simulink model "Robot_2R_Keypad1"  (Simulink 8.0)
settings: Solver=ode3  StartTime=0.0  StopTime=inf  RelTol=1e-3
InitFcn:
  | dt=0.01;
  | Kp=400; Kd=0; Ki=0;
undefined symbols (not defined in the file or in its folder): DiscIntNeverNeededParam
libraries: arduinolib x9, simulink x2

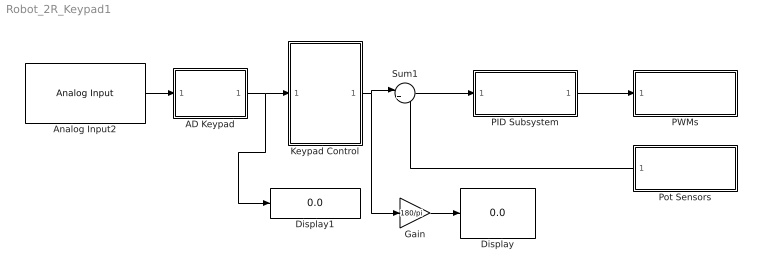
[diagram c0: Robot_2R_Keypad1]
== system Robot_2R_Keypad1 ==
  AD Keypad : MATLAB Function  TreatAsAtomicUnit=on
  Analog Input2 : arduinolib/Analog Input  pinNumber=2  sampleTime=dt
  Display : Display
  Display1 : Display
  Gain : Gain  Gain=180/pi
  Keypad Control : MATLAB Function  TreatAsAtomicUnit=on
  PID Subsystem : Subsystem  TreatAsAtomicUnit=on
  PWMs : Subsystem  TreatAsAtomicUnit=on
  Pot Sensors : Subsystem  TreatAsAtomicUnit=on
  Sum1 : Sum  Inputs=|+-
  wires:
  PID Subsystem/1(Out1) -> PWMs/1(In1)
  Sum1/1 -> PID Subsystem/1(In1)
  Pot Sensors/1(Out1) -> Sum1/2
  Analog Input2/1 -> AD Keypad/1(u)
  AD Keypad/1(y) -> Display1/1, Keypad Control/1(key)
  Keypad Control/1(thd) -> Gain/1, Sum1/1
  Gain/1 -> Display/1

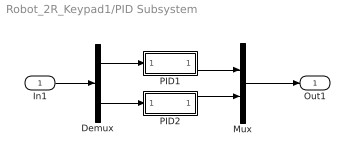
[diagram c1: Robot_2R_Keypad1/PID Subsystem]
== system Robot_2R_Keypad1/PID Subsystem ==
  In1 : Inport
  Demux : Demux  Outputs=2
  Mux : Mux  Inputs=2
  PID1 : Subsystem
  PID2 : Subsystem
  Out1 : Outport
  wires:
  In1/1 -> Demux/1
  Demux/1 -> PID1/1(In1)
  PID1/1(Out1) -> Mux/1
  Demux/2 -> PID2/1(In1)
  PID2/1(Out1) -> Mux/2
  Mux/1 -> Out1/1

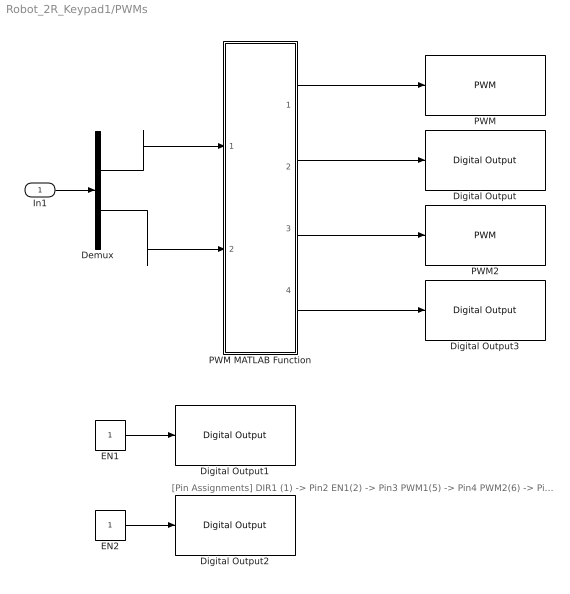
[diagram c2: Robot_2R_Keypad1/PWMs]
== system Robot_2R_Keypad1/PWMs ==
  note: [Pin Assignments] DIR1 (1) -> Pin2 EN1(2) -> Pin3 PWM1(5) -> Pin4 PWM2(6) -> Pin5 DIR2 (7) -> Pin6 EN2(8) -> Pin7
  In1 : Inport
  Demux : Demux  Outputs=2
  Digital Output : arduinolib/Digital Output  pinNumber=2
  Digital Output1 : arduinolib/Digital Output  pinNumber=3
  Digital Output2 : arduinolib/Digital Output  pinNumber=7
  Digital Output3 : arduinolib/Digital Output  pinNumber=6
  EN1 : Constant
  EN2 : Constant
  PWM : arduinolib/PWM  pinNumber=4
  PWM MATLAB Function : MATLAB Function  TreatAsAtomicUnit=on
  PWM2 : arduinolib/PWM  pinNumber=5
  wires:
  EN1/1 -> Digital Output1/1
  EN2/1 -> Digital Output2/1
  In1/1 -> Demux/1
  Demux/1 -> PWM MATLAB Function/1(u1)
  Demux/2 -> PWM MATLAB Function/2(u2)
  PWM MATLAB Function/1(pwm1) -> PWM/1
  PWM MATLAB Function/2(dir1) -> Digital Output/1
  PWM MATLAB Function/3(pwm2) -> PWM2/1
  PWM MATLAB Function/4(dir2) -> Digital Output3/1

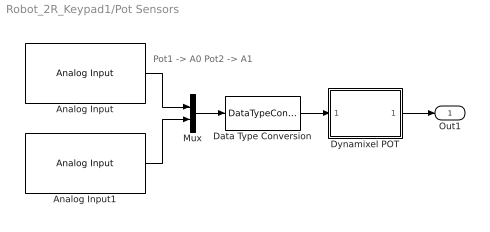
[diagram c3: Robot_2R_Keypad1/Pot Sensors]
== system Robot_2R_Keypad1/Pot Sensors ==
  note: Pot1 -> A0 Pot2 -> A1
  Analog Input : arduinolib/Analog Input  pinNumber=0  sampleTime=dt
  Analog Input1 : arduinolib/Analog Input  pinNumber=1  sampleTime=dt
  Data Type Conversion : DataTypeConversion  OutDataTypeStr=double
  Dynamixel POT : MATLAB Function  TreatAsAtomicUnit=on
  Mux : Mux  Inputs=2
  Out1 : Outport
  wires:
  Analog Input/1 -> Mux/1
  Analog Input1/1 -> Mux/2
  Mux/1 -> Data Type Conversion/1
  Data Type Conversion/1 -> Dynamixel POT/1(u)
  Dynamixel POT/1(y) -> Out1/1

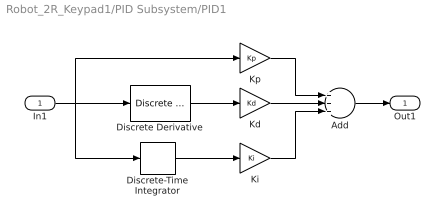
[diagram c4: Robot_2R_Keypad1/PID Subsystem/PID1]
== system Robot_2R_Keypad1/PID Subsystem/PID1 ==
  In1 : Inport
  Add : Sum  Inputs=+++
  Discrete Derivative : simulink/Discrete/Discrete Derivative  gainval=1.0  ICPrevScaledInput=0.0  InputProcessing=Inherited  OutMin=[]  OutMax=[]  OutDataType=fixdt(1, 16)  OutScaling=2^-10  DoSatur=off
  Discrete-Time Integrator : DiscreteIntegrator  SampleTime=dt  ICPrevOutput=DiscIntNeverNeededParam  ICPrevScaledInput=DiscIntNeverNeededParam
  Kd : Gain  Gain=Kd
  Ki : Gain  Gain=Ki
  Kp : Gain  Gain=Kp
  Out1 : Outport
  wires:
  Discrete-Time Integrator/1 -> Ki/1
  Kp/1 -> Add/1
  Kd/1 -> Add/2
  Ki/1 -> Add/3
  Discrete Derivative/1 -> Kd/1
  Add/1 -> Out1/1
  In1/1 -> Kp/1, Discrete Derivative/1, Discrete-Time Integrator/1

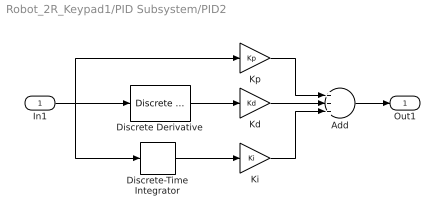
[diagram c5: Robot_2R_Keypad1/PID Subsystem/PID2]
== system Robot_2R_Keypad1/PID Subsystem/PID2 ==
  In1 : Inport
  Add : Sum  Inputs=+++
  Discrete Derivative : simulink/Discrete/Discrete Derivative  gainval=1.0  ICPrevScaledInput=0.0  InputProcessing=Inherited  OutMin=[]  OutMax=[]  OutDataType=fixdt(1, 16)  OutScaling=2^-10  DoSatur=off
  Discrete-Time Integrator : DiscreteIntegrator  SampleTime=dt  ICPrevOutput=DiscIntNeverNeededParam  ICPrevScaledInput=DiscIntNeverNeededParam
  Kd : Gain  Gain=Kd
  Ki : Gain  Gain=Ki
  Kp : Gain  Gain=Kp
  Out1 : Outport
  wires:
  Discrete-Time Integrator/1 -> Ki/1
  Kp/1 -> Add/1
  Kd/1 -> Add/2
  Ki/1 -> Add/3
  Discrete Derivative/1 -> Kd/1
  Add/1 -> Out1/1
  In1/1 -> Kp/1, Discrete Derivative/1, Discrete-Time Integrator/1

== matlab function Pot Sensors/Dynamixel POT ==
function y = fcn(u)

MAX_CH=2;
y=zeros(MAX_CH,1);

for ch=1:MAX_CH
    y(ch,1)=(pi/180)*(300/1024)*(u(ch,1)-204.8);
end

== matlab function PWMs/PWM
MATLAB Function ==
function [pwm1, dir1, pwm2, dir2] = fcn(u1, u2)

if u1>=0,dir1=1;
else dir1=0; end

if u2>=0,dir2=1;    
else dir2=0; end

pwm1=abs(u1);
pwm2=abs(u2);
% Saturation %
if pwm1>=255, pwm1=255; end
if pwm2>=255, pwm2=255; end

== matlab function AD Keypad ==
function y = fcn(u)
y=-1;
if u>=0 && u<(64-32), y=0; end
if u>=(64-32) && u<(64+32), y=1; end
if u>=(128-32) && u<(128+32), y=2; end
if u>=(192-32) && u<(192+32), y=3; end
if u>=(256-32) && u<(256+32), y=4; end
if u>=(320-32) && u<(320+32), y=5; end
if u>=(384-32) && u<(384+32), y=6; end
if u>=(448-32) && u<(448+32), y=7; end
if u>=(512-32) && u<(512+32), y=8; end
if u>=(576-32) && u<(576+32), y=9; end
if u>=(640-32) && u<(640+32), y=10; end
if u>=(704-32) && u<(704+32), y=11; end
if u>=(768-32) && u<(768+32), y=12; end
if u>=(832-32) && u<(832+32), y=13; end
if u>=(896-32) && u<(896+32), y=14; end
if u>=(960-32) && u<(960+32), y=15; end
if u<0 || u>=(960+32), y=-1; end

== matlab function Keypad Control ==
function thd = fcn(key)

persistent x_p th_p
 
D2R=pi/180;
dpos=0.5; dth=0.5*D2R;
a1=	45; a2=45;
param=[0,a1,0; 0,a2,0];
 
if isempty(x_p), x_p=[a1,a2]'; end
if isempty(th_p), th_p=[0,90*D2R]'; end

% Init 
th=th_p; x=x_p;
 
switch key
    case 0, th(1,1)=th_p(1,1)+dth; index=1;        % +th1 Movement %
    case 4, th(1,1)=th_p(1,1)-dth; index=1;        % -th1 Movement %
    case 1, th(2,1)=th_p(2,1)+dth; index=1;        % +th2 Movement %
    case 5, th(2,1)=th_p(2,1)-dth; index=1;        % -th2 Movement %              
 
    case 2, x(1,1)=x_p(1,1)+dpos; index=2;      % +X Movement %
    case 6, x(1,1)=x_p(1,1)-dpos; index=2;      % -X Movement %
    case 3, x(2,1)=x_p(2,1)+dpos; index=2;      % +Y Movement %
    case 7, x(2,1)=x_p(2,1)-dpos; index=2;      % -Y Movement %   
        
    case 15, x=[a1,a2]'; th=[0,90*D2R]'; index=1;   % Original Pos & Orien %        
    otherwise
        th=th_p; index=1;
end
 
switch index
    case 1, % Forward Kinematics %
        if (th(1,1)<-30*D2R || th(1,1)>=D2R*210) || (th(2,1)<-30*D2R || th(2,1)>=D2R*210),
            th=th_p;
        end        
        T02=forward_kinematics(th, param);
        x=T02(1:2,4);
    case 2, % Inverse Kinematics %
        if (x(1,1)<-(a1+a2) || x(1,1)>+(a1+a2)) || (x(2,1)<-0.5*a1 || x(2,1)>+(a1+a2))
            x=x_p;
        end
        
        [th_c, w_index]=inverse_kinematics(x, param);
        if w_index==1, th=th_c; end
end

thd=th;

% Back substitution %
th_p=th; x_p=x;

%-------- Forward Kinematics
function T=forward_kinematics(th, param)
T=Transformation(th(1,1), param(1,:))*Transformation(th(2,1), param(2,:));
 
%-------- Inverse Kinematics
function [th, w_index]=inverse_kinematics(pos, param)
w_index=1;  % In workspace %
a1=param(1,2); a2=param(2,2);
 
% (1) Calculate th2 %
px=pos(1,1); py=pos(2,1);
kapha=(px^2+py^2-a1^2-a2^2)/(2*a1*a2);
if abs(kapha)>1
    w_index=-1;  % Out of Workspace %
    kapha=1;
end
th2=+acos(kapha); % Elbow Down %
%th2=-acos(kapha); % Elbow Up %
 
% (2) Calculate th1 %
delta=a1^2+a2^2+2*a1*a2*cos(th2);
cth1=(px*(a1+a2*cos(th2))+py*a2*sin(th2))/delta;
sth1=(-px*a2*sin(th2)+py*(a1+a2*cos(th2)))/delta;
th1=atan2(sth1, cth1); 
th=[th1, th2]';
 
%-------- D-H Transformation Matrix
function [T]=Transformation(th, param)
alpha=param(1); a=param(2); d=param(3);
T=Trans([0,0,d]')*Rotz(th)*Trans([a,0,0]')*Rotx(alpha);

%------- Rotation matrix about the X-axis 
function [T]=Rotx(th)
cx=cos(th); sx=sin(th);
T=[1,0,0,0; 0,cx,-sx,0; 0,sx,cx,0; 0,0,0,1];
 
%------- Rotation matrix about the Z-axis 
function [T]=Rotz(th)
cz=cos(th); sz=sin(th);
T=[cz,-sz,0,0; sz,cz,0,0; 0,0,1,0; 0,0,0,1];
 
%-------- Translation along the x, y, z axes 
function [T]=Trans(p)
T=[1,0,0,p(1,1); 0,1,0,p(2,1); 0,0,1,p(3,1); 0,0,0,1];
